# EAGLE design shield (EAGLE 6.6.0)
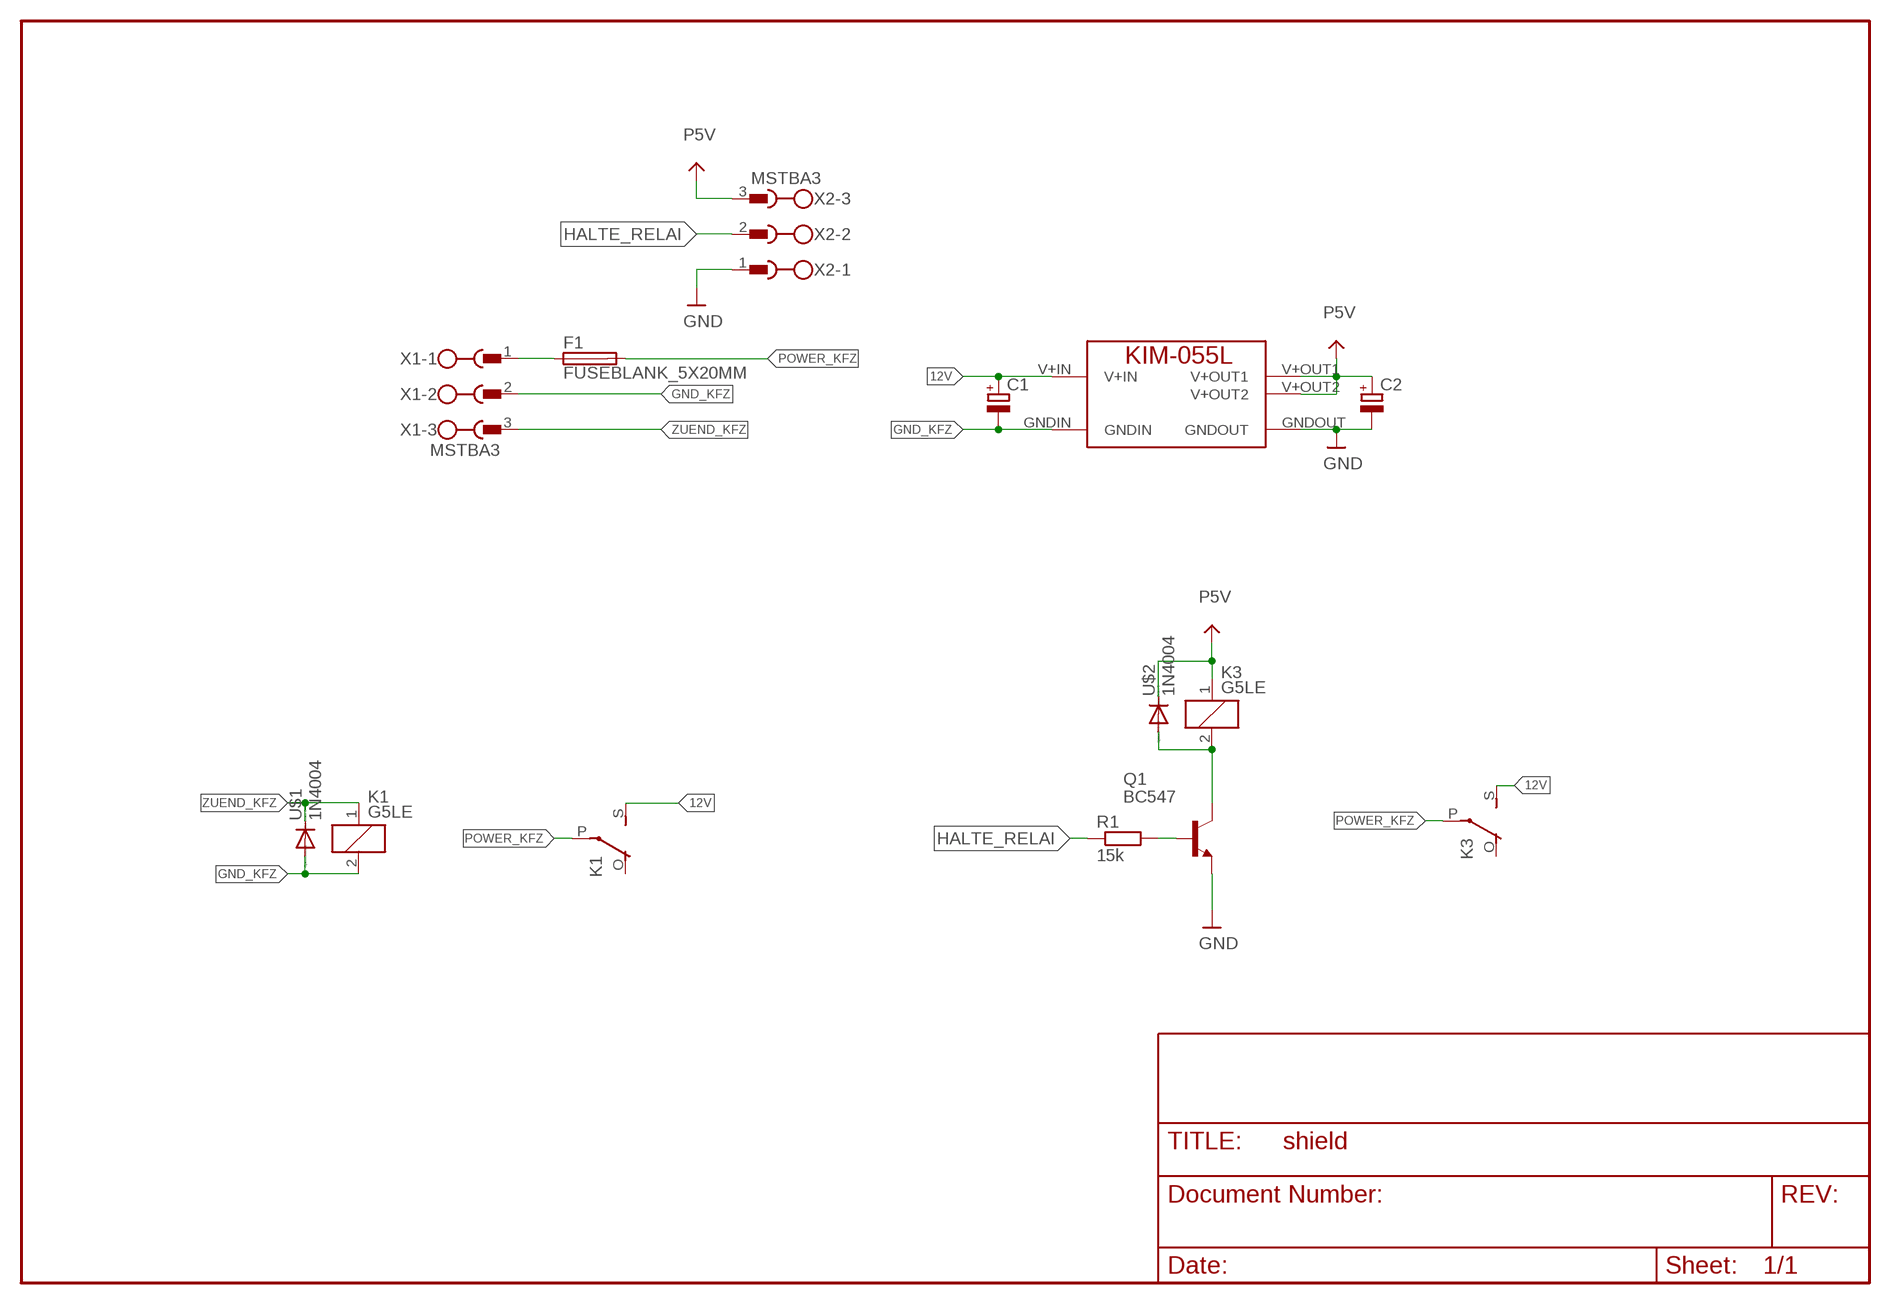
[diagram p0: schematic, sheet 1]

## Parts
C1  CPOL-EUE5-13  [E5-13]
C2  CPOL-EUE5-13  [E5-13]
F1  FUSEBLANK_5X20MM  [FUSE_HOLDER_5X20MM]
K1  G5LE  [G5LE]
K3  G5LE  [G5LE]
MOD1  KIM-055L  [KIM-055L]
Q1  BC547  [TO92]
R1  15k  R-EU_0207/7  [0207/7]
U$1  1N4004  [DO41-10]
U$2  1N4004  [DO41-10]
X1  MSTBA3  [MSTBA3]
X2  MSTBA3  [MSTBA3]

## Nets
12V: C1.+ K1.S(2:S) K3.S(2:S) MOD1.V+IN
GND: C2.- MOD1.GNDOUT Q1.1(E) X2.1
GND_KFZ: C1.- K1.2 MOD1.GNDIN U$1.A X1.2
HALTE_RELAI: R1.1 X2.2
N$1: K3.2 Q1.3(C) U$2.A
N$2: Q1.2(B) R1.2
N$3: F1.1 X1.1
P5V: C2.+ K3.1 MOD1.V+OUT1 MOD1.V+OUT2 U$2.C X2.3
POWER_KFZ: F1.2 K1.P(2:P) K3.P(2:P)
ZUEND_KFZ: K1.1 U$1.C X1.3
Unconnected: K1.O(2:O) K3.O(2:O)

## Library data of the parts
C1 C2 = schlager_passiv:CPOL-EU: POLARIZED CAPACITOR, European symbol
F1 = fuse:FUSE: Fuse; OC_FARNELL: unknown; OC_NEWARK: unknown
K1 K3 = relay:G5LE: RELAY 1 x switch, 10 A/120 V AC, 8 A/30 V DC, Omron; OC_FARNELL: unknown; OC_NEWARK: unknown
MOD1 = kim055l:KIM-055L: 5V 5amp DC DC module. IMPORANT: Add low ESR input & output capacitors. V+OUT1 & V+OUT2 internally connected.
Q1 = transistor-npn:BC547*: NPN Transistor
R1 = schlager_passiv:R-EU_: RESISTOR, European symbol
U$1 U$2 = diode:1N4004: DIODE
X1 X2 = X_Phoenix:MSTBA3: PHOENIX

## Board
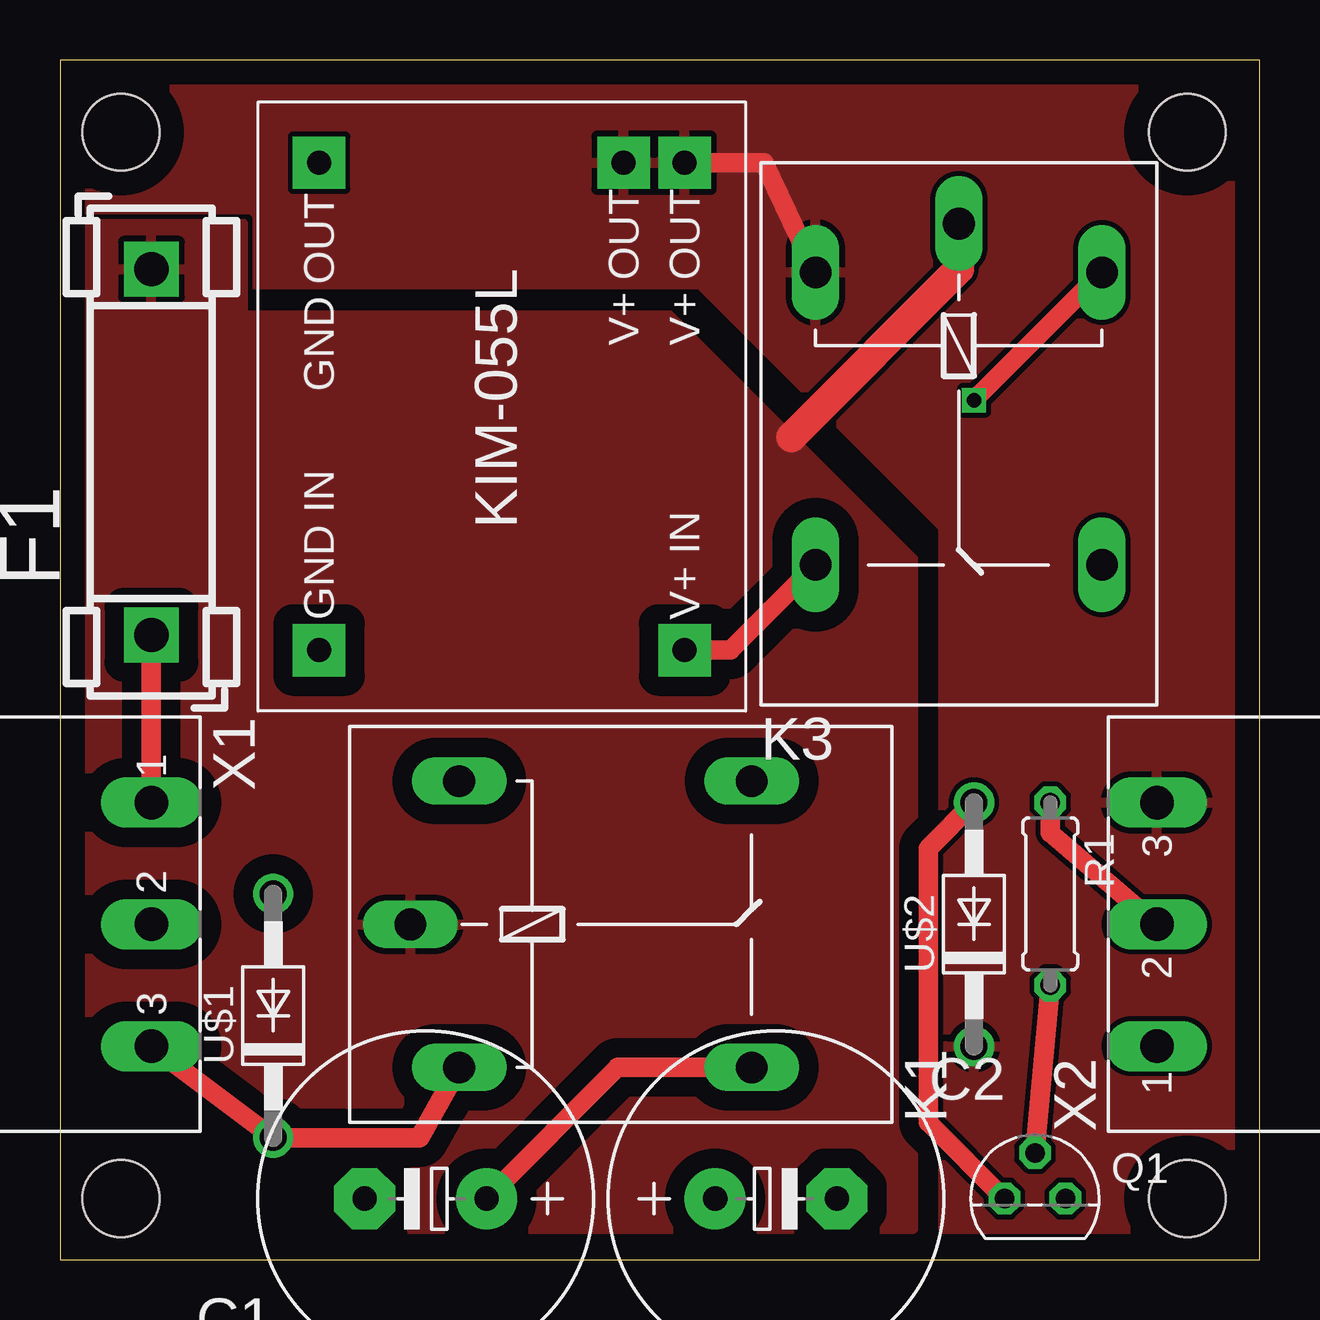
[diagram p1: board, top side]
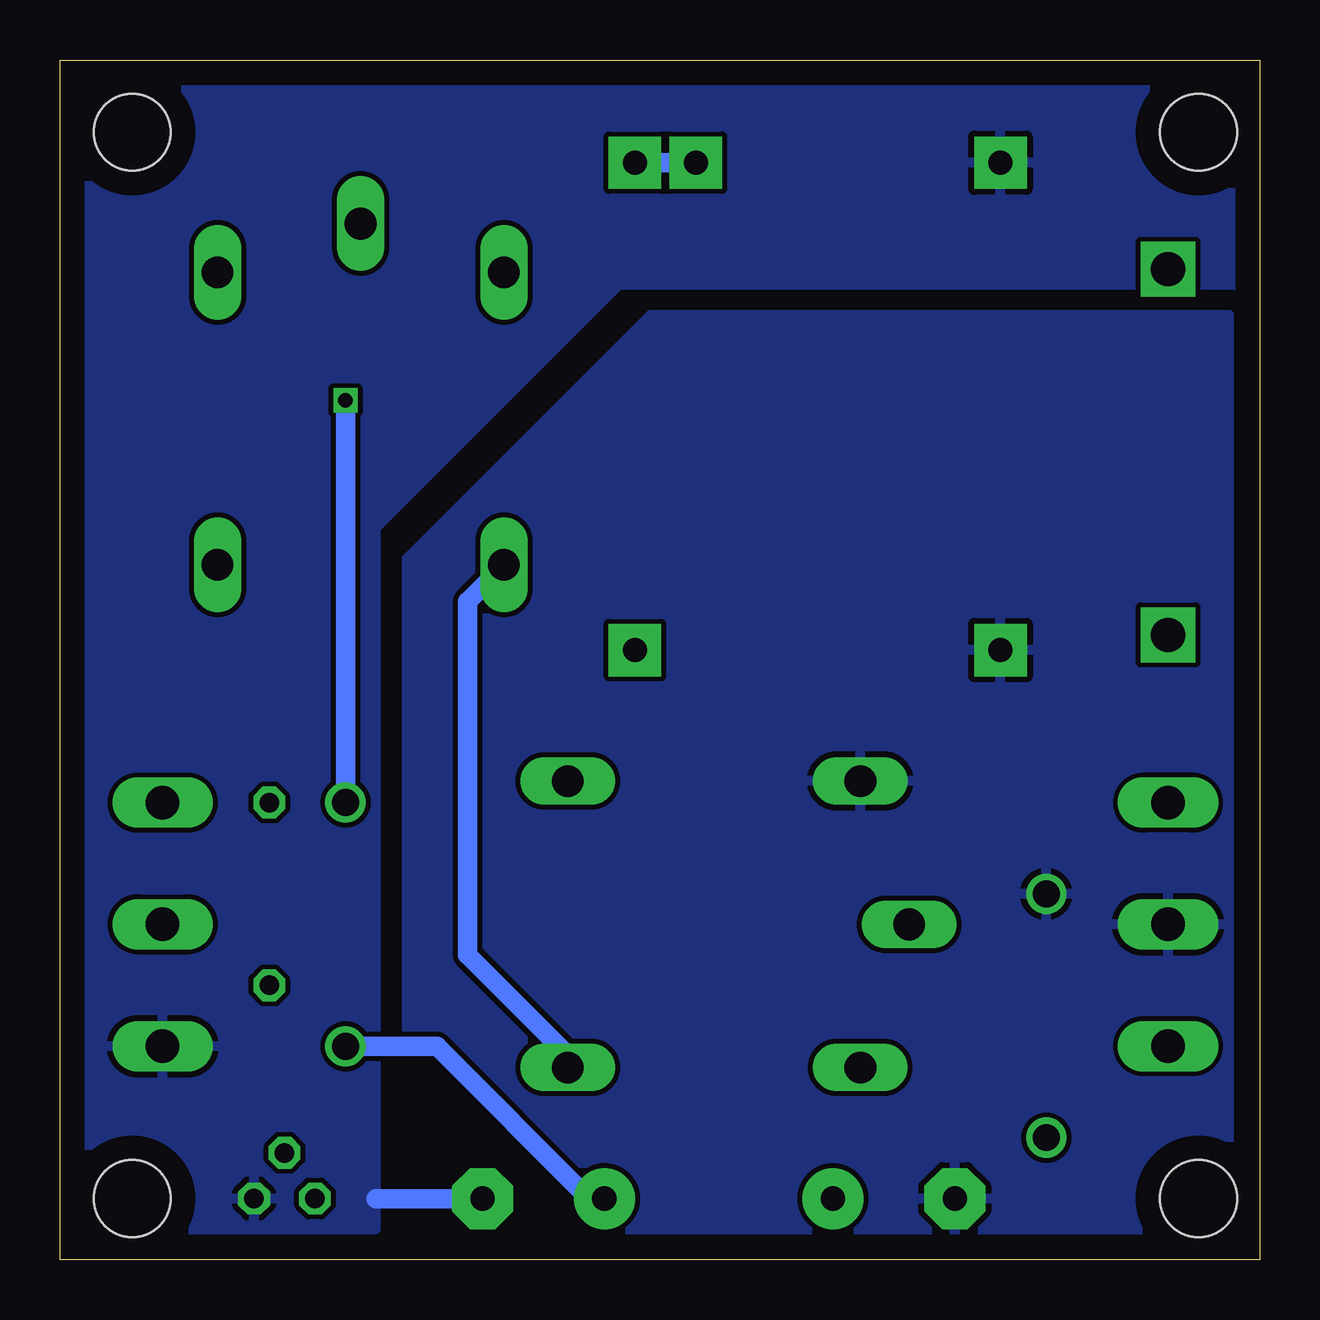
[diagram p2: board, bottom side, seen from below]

Size 50 x 50 mm. Coordinates in mm from the lower left corner, seen from the top.
Outline: 0,0 50,0 50,50 0,50 0,0
Copper layers (1*16): Top 0.035mm / dielectric 1.5mm / Bottom 0.035mm
Design rules "default": minimum track width 10mil, minimum drill 24mil, track to track 8mil, track to pad 8mil, pad to pad 8mil, via to via 8mil, smd to smd 8mil, copper to edge 40mil, drill to drill 8mil, minimum pad ring 10mil, minimum via ring 8mil, stop-mask expansion 4mil, vias tented up to drill 0mil, thermal gap 10mil
Holes 3.2 mm at 2.54,2.54 46.99,2.54 46.99,46.99 2.54,46.99

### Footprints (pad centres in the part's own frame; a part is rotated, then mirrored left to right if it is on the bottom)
E5-13 = drill 1.016 pad 2.54: + -2.54,0 | drill 1.016 pad 2.54 octagon: - 2.54,0
FUSE_HOLDER_5X20MM = drill 1.422 pad 2.286 square: 1 0,0; 2 15.24,0
G5LE = drill 1.321 long: 1 -7.493,-5.969; 2 -7.493,5.969; O 4.699,5.969; P -9.525,0; S 4.699,-5.969
KIM-055L = drill 1 pad 2.184 square: GNDIN -10.16,7.62; GNDOUT 10.16,7.62; V+IN -10.16,-7.62; V+OUT1 10.16,-5.08; V+OUT2 10.16,-7.62
TO92 = drill 0.813 octagon: 1 1.27,0; 2 0,1.905; 3 -1.27,0
0207/7 = drill 0.813 octagon: 1 -3.81,0; 2 3.81,0
DO41-10 = drill 1.118: A 5.08,0; C -5.08,0
MSTBA3 = drill 1.397 long: 1 -5.08,5.08; 2 0,5.08; 3 5.08,5.08

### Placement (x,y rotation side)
C1  15.24,2.54 180 top
C2  29.84,2.54 0 top
F1  3.81,26.04 90 top
K1  24.13,13.97 0 top
K3  37.47,33.66 270 top
MOD1  18.41,35.56 90 top
Q1  40.64,2.54 0 top
R1  41.27,15.24 270 top
U$1  8.89,10.16 90 top
U$2  38.1,13.97 90 top
X1  -1.27,13.97 270 top
X2  50.8,13.97 90 top

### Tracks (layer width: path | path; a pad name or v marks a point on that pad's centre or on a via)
12V
  Top 0.813: K3.S 27.94,25.4 MOD1.V+IN | K1.S 23.24,8 C1.+
  Bottom 0.813: K1.S 28.83,8.51 33.02,12.7 33.02,27.43 K3.S
GND
  Bottom 0.813: C2.- 36.83,2.54
  pour Bottom: 0,49.53 49.53,49.53 49.53,1.27 36.83,1.27 36.83,30.48 26.67,40.64 0,40.64
GND_KFZ
  pour Bottom: 1.27,39.37 25.4,39.37 35.56,29.21 35.56,1.27 1.27,1.27
HALTE_RELAI
  Top 0.813: X2.2 41.27,17.78 R1.1
N$1  (via drill 0.6)
  Top 0.813: Q1.3 36.2,5.71 36.2,17.14 U$2.A | v38.1,35.81 K3.2
  Bottom 0.813: U$2.A v38.1,35.81
N$2
  Top 0.813: R1.2 Q1.2
N$3
  Top 0.813: X1.1 F1.1
P5V
  Top 0.813: MOD1.V+OUT2 29.34,45.72 K3.1
  Bottom 0.813: MOD1.V+OUT2 MOD1.V+OUT1 | C2.+ 27.94,2.54 34.29,8.89 U$2.C
  pour Top (rank 6): 0,49.53 49.53,49.53 49.53,1.27 36.83,1.27 36.83,30.48 26.67,40.64 0,40.64
POWER_KFZ
  Top 1.27: K3.P 37.47,41.27 30.48,34.29
  pour Top (isolate 0.813, rank 3): 1.27,1.27 1.27,43.18 7.62,43.18 7.62,39.37 25.4,39.37 35.56,29.21 35.56,1.27
ZUEND_KFZ
  Top 0.813: K1.1 14.99,5.08 U$1.C X1.3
